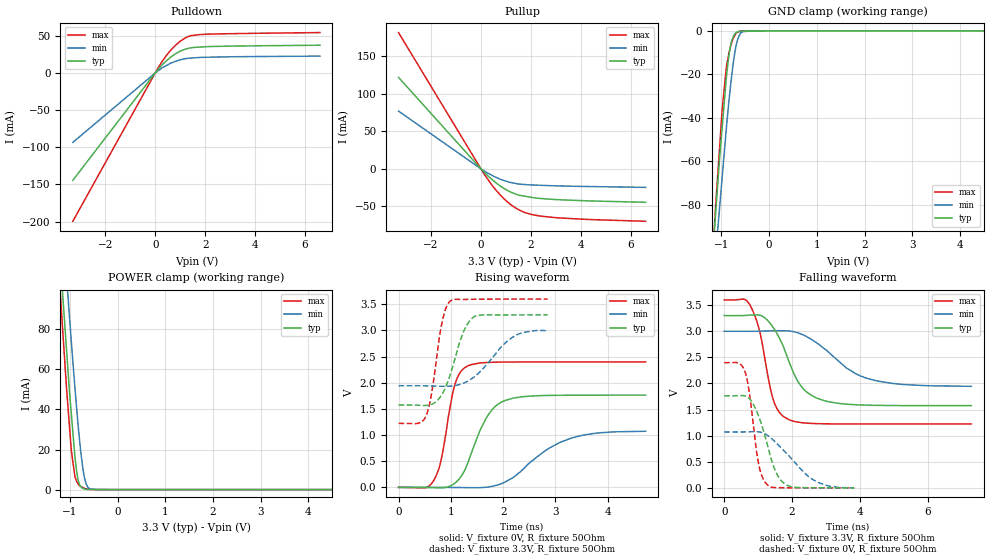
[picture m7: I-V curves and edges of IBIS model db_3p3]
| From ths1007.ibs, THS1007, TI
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|   db_3p3 Model
[Model]   db_3p3
Model_type   I/O
Polarity   Non-Inverting
Enable   Active-High
Vinl = 0.6
Vinh = 2
Vmeas = 1.65
Vref = 1.65
Cref = 30pF
Rref = 50
|   typ   min   max
|   (nom PVT)   (fast PVT)   (slow PVT)
C_comp   1.853e-12   1.842e-12   1.894e-12
|ON state : BUFFER OUTPUT TURNED HIGH
|C_comp   1.967e-12   1.956e-12   2.023e-12
|OFF state: BUFFER IN HIGH IMPEDANCE
|C_comp   1.738e-12   1.729e-12   1.765e-12
| Where nom  PVT is Nominal Process, 3.3V, 27C
| Fast PVT is Strong Process,  3.6V, -40C
| Slow PVT is Weak Process,   3V, 125C
[Voltage Range]   3.3   3   3.6
|Ambient Temperature   25   85   -40
|Junction Temperature
[Temperature Range]   27   125   -40
[Pullup Reference]   3.3   3   3.6
[Pulldown Reference]   0   0   0
[Power Clamp Reference]   3.3   3   3.6
[GND Clamp Reference]   0   0   0
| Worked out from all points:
|   slope of the pulldown table from 0 to 0.495 V, typ, clamps not added: 28 ohm
|   slope of the pullup table from 0 to 0.495 V, typ, clamps not added: 31.6 ohm
|   GND clamp passes 1 mA (typ) near -0.70 V on its own axis
|   POWER clamp passes 1 mA (typ) near -0.75 V on its own axis
|   falling waveform, V_fixture 3.3V, R_fixture 50Ohm: 20-80 % time 741ps typ, 1.27ns min, 450ps max; typ from 3.3 V to 1.58 V
|   rising waveform, V_fixture 0V, R_fixture 50Ohm: 20-80 % time 455ps typ, 859ps min, 261ps max; typ from 0 V to 1.76 V
|   rising waveform, V_fixture 3.3V, R_fixture 50Ohm: 20-80 % time 333ps typ, 571ps min, 212ps max; typ from 1.58 V to 3.3 V
|   falling waveform, V_fixture 0V, R_fixture 50Ohm: 20-80 % time 500ps typ, 950ps min, 292ps max; typ from 1.76 V to 0 V
[Pulldown]
|   Voltage   I(typ)   I(min)   I(max)
-3.3V     -144.5mA   -93.38mA   -199.6mA
154.8mV   6.391mA    3.9mA      9.041mA
424.8mV   15.59mA    9.622mA    22.52mA
630mV     21.64mA    13.42mA    30.96mA
1.008V    29.35mA    17.89mA    42.82mA
1.35V     33.32mA    19.96mA    49.36mA
1.836V    34.94mA    21.01mA    51.79mA
6.6V      37.38mA    22.72mA    54.4mA
[GND Clamp]
|   Voltage   I(typ)   I(min)   I(max)
-3.3V     -899.5mA   -841.1mA   -977.4mA
-1.234V   -119.1mA   -136.4mA   -122.1mA
-1.123V   -84.79mA   -104.8mA   -81.36mA
-1.065V   -66.81mA   -88.23mA   -62.42mA
-986.4mV  -45.04mA   -67.97mA   -36.97mA
-896.4mV  -21.57mA   -44.78mA   -16.66mA
-858mV    -13.91mA   -35.86mA   -12.06mA
-785.4mV  -4.717mA   -20.8mA    -5.47mA
-708mV    -1.258mA   -8.591mA   -1.732mA
-620.4mV  -156.6uA   -1.956mA   -275.6uA
-285mV    -71.48uA   -357.5nA   -115.2nA
6.6V      0A         0A         0A
[Pullup]
|   Voltage   I(typ)   I(min)   I(max)
-3.3V     122.1mA    77.06mA    181.9mA
172.8mV   -6.009mA   -3.688mA   -9.119mA
633.6mV   -19.54mA   -11.88mA   -29.75mA
918mV     -26.02mA   -15.65mA   -39.85mA
1.145V    -30.21mA   -17.93mA   -46.49mA
1.382V    -33.59mA   -19.49mA   -52.13mA
1.706V    -36.31mA   -20.85mA   -57.68mA
2.012V    -38.04mA   -21.53mA   -60.82mA
2.473V    -39.84mA   -22.12mA   -63.46mA
4.162V    -42.64mA   -23.56mA   -67.44mA
6.6V      -44.7mA    -24.77mA   -70.09mA
[POWER Clamp]
|   Voltage   I(typ)   I(min)   I(max)
-3.3V     946.7mA    946.9mA    966.3mA
-1.227V   123.3mA    159mA      106.9mA
-1.188V   109.1mA    145.5mA    92.22mA
-1.076V   71.14mA    107.9mA    51.98mA
-1.038V   58.09mA    95mA       39.96mA
-972mV    37.88mA    73.74mA    19.51mA
-861.3mV  9.211mA    40.83mA    4.177mA
-792mV    2.047mA    22.92mA    1.77mA
-726mV    538.3uA    9.896mA    988.8uA
-627mV    83.82uA    1.247mA    270.5uA
-399mV    53.18uA    2.449uA    499.6nA
6.6V      0A         0A         0A
[Ramp]
R_load = 50
|   typ   min   max
dV/dt_r   1.0583/4.54011e-10   0.642088/8.52145e-10   1.43898/2.60429e-10
dV/dt_f   1.03457/7.40338e-10   0.633907/1.27722e-09   1.42547/4.47967e-10
[Falling Waveform]
V_fixture = 3.3V
V_fixture_min = 3V
V_fixture_max = 3.6V
R_fixture = 50Ohm
|   Time   V(typ)   V(min)   V(max)
0s        3.3V       3V         3.6V
760ps     3.309V     3V         3.5V
1.04ns    3.309V     3.001V     3.016V
1.45ns    3.066V     3.009V     1.681V
1.915ns   2.408V     3.005V     1.304V
2.305ns   1.915V     2.936V     1.247V
3.03ns    1.657V     2.625V     1.227V
3.9ns     1.592V     2.178V     1.224V
4.53ns    1.58V      2.046V     1.224V
7.285ns   1.576V     1.945V     1.224V
[Rising Waveform]
V_fixture = 0V
V_fixture_min = 0V
V_fixture_max = 0V
R_fixture = 50Ohm
|   Time   V(typ)   V(min)   V(max)
0s        1.442nV    2.279nV    1.234nV
515ps     -1.14mV    195.1uV    -8.794mV
680ps     -5.557mV   241.8uV    143mV
820ps     -9.361mV   -78.03uV   549.9mV
1.07ns    75.14mV    -2.105mV   1.938V
1.325ns   465mV      -5.553mV   2.323V
1.675ns   1.321V     2.415mV    2.387V
2.04ns    1.663V     102.4mV    2.396V
3.305ns   1.762V     942.8mV    2.398V
4.725ns   1.764V     1.073V     2.398V
[Rising Waveform]
V_fixture = 3.3V
V_fixture_min = 3V
V_fixture_max = 3.6V
R_fixture = 50Ohm
|   Time   V(typ)   V(min)   V(max)
0s        1.576V     1.943V     1.224V
380ps     1.571V     1.943V     1.225V
525ps     1.567V     1.942V     1.362V
635ps     1.589V     1.939V     1.813V
835ps     1.785V     1.933V     3.168V
1.005ns   2.206V     1.937V     3.575V
1.245ns   2.981V     1.994V     3.594V
1.445ns   3.262V     2.112V     3.597V
2.165ns   3.297V     2.862V     3.6V
2.85ns    3.3V       2.997V     3.6V
[Falling Waveform]
V_fixture = 0V
V_fixture_min = 0V
V_fixture_max = 0V
R_fixture = 50Ohm
|   Time   V(typ)   V(min)   V(max)
0s        1.764V     1.07V      2.398V
425ps     1.766V     1.07V      2.392V
615ps     1.762V     1.071V     2.22V
735ps     1.715V     1.073V     1.844V
1ns       1.397V     1.074V     509.3mV
1.25ns    877.2mV    1.017V     72.87mV
1.545ns   275.5mV    852.8mV    4.884mV
1.88ns    42.22mV    630.5mV    1.575mV
2.73ns    1.762mV    114.5mV    221uV
3.83ns    253.1uV    484.6uV    128.9uV
